FUNCTION_BLOCK FB112
TITLE =Set Velocity Must
//*****************************************************************************
//* maxon motor ag
//* R&D
//* all rights reserved
//*****************************************************************************
//* Summary:  Write demand value of velocity
//*
//* Remarks:
//*
//* Created under: STEP7 REV5.2+SP1
//*****************************************************************************
//* History:
//* 18.05.2004 | INA   first release
//*
//*
//*****************************************************************************
//

AUTHOR:INA
FAMILY:Velocity
NAME:SetVeloM
VERSION:00.01


VAR_INPUT

Write : BOOL //A rising edge start the command

  NodeID : BYTE //Adress of the maxon device

  VelocityMust : DINT //Velocity demand value

END_VAR
VAR_OUTPUT
  Done : BOOL //Data valid flag is TRUE if data were available

  Err : BOOL //Error flag is TRUE if an Error has occured, see ErrNo for more details

  ErrNo : DINT //Contains detailed error information

END_VAR
VAR
  xEdgeMerker : BOOL //Edge Merker

  xEdgeFlag : BOOL //Edge Flag

  xStep : INT
END_VAR

BEGIN

NETWORK
TITLE = Activate the service function
//

// SDO Write "Set Velocity Must"

       U    #Write
       FP   #xEdgeFlag                   // recognize a positiv edge of the Read signal
       =    #xEdgeMerker                 // and set the xEdgeMerker for one cycle to true

       L    #xStep
       L    0
       ==I
       U    #xEdgeMerker
       SPB  nstp                         // iStep = 1 -> fnc1

       L    #xStep                       // jump list
       SPL  List
       SPA  rdef
       SPA  fnc1
       SPA  fncE
List  :SPA  rdef

rdef  :NOP  0
       R    #Done                        // reset Done
       R    #Err
       L    0
       T    #xStep                       // iStep = 0
       SPA  end

fnc1  :NOP  0
       CALL FC13
         NodeID:=#NodeID
         Index:=DW#16#0000206B
         SubIndex:=DW#16#00000000
         ValueIn:=#VelocityMust
         RET_VAL:=#Done
         Err:=#Err
         ErrNo:=#ErrNo

fncE  :NOP  0
       L    0
       T    #xStep
       SPA  end

nstp  :NOP  0
       L    #xStep
       INC            1
       T    #xStep

end   :NOP  0
END_FUNCTION_BLOCK
